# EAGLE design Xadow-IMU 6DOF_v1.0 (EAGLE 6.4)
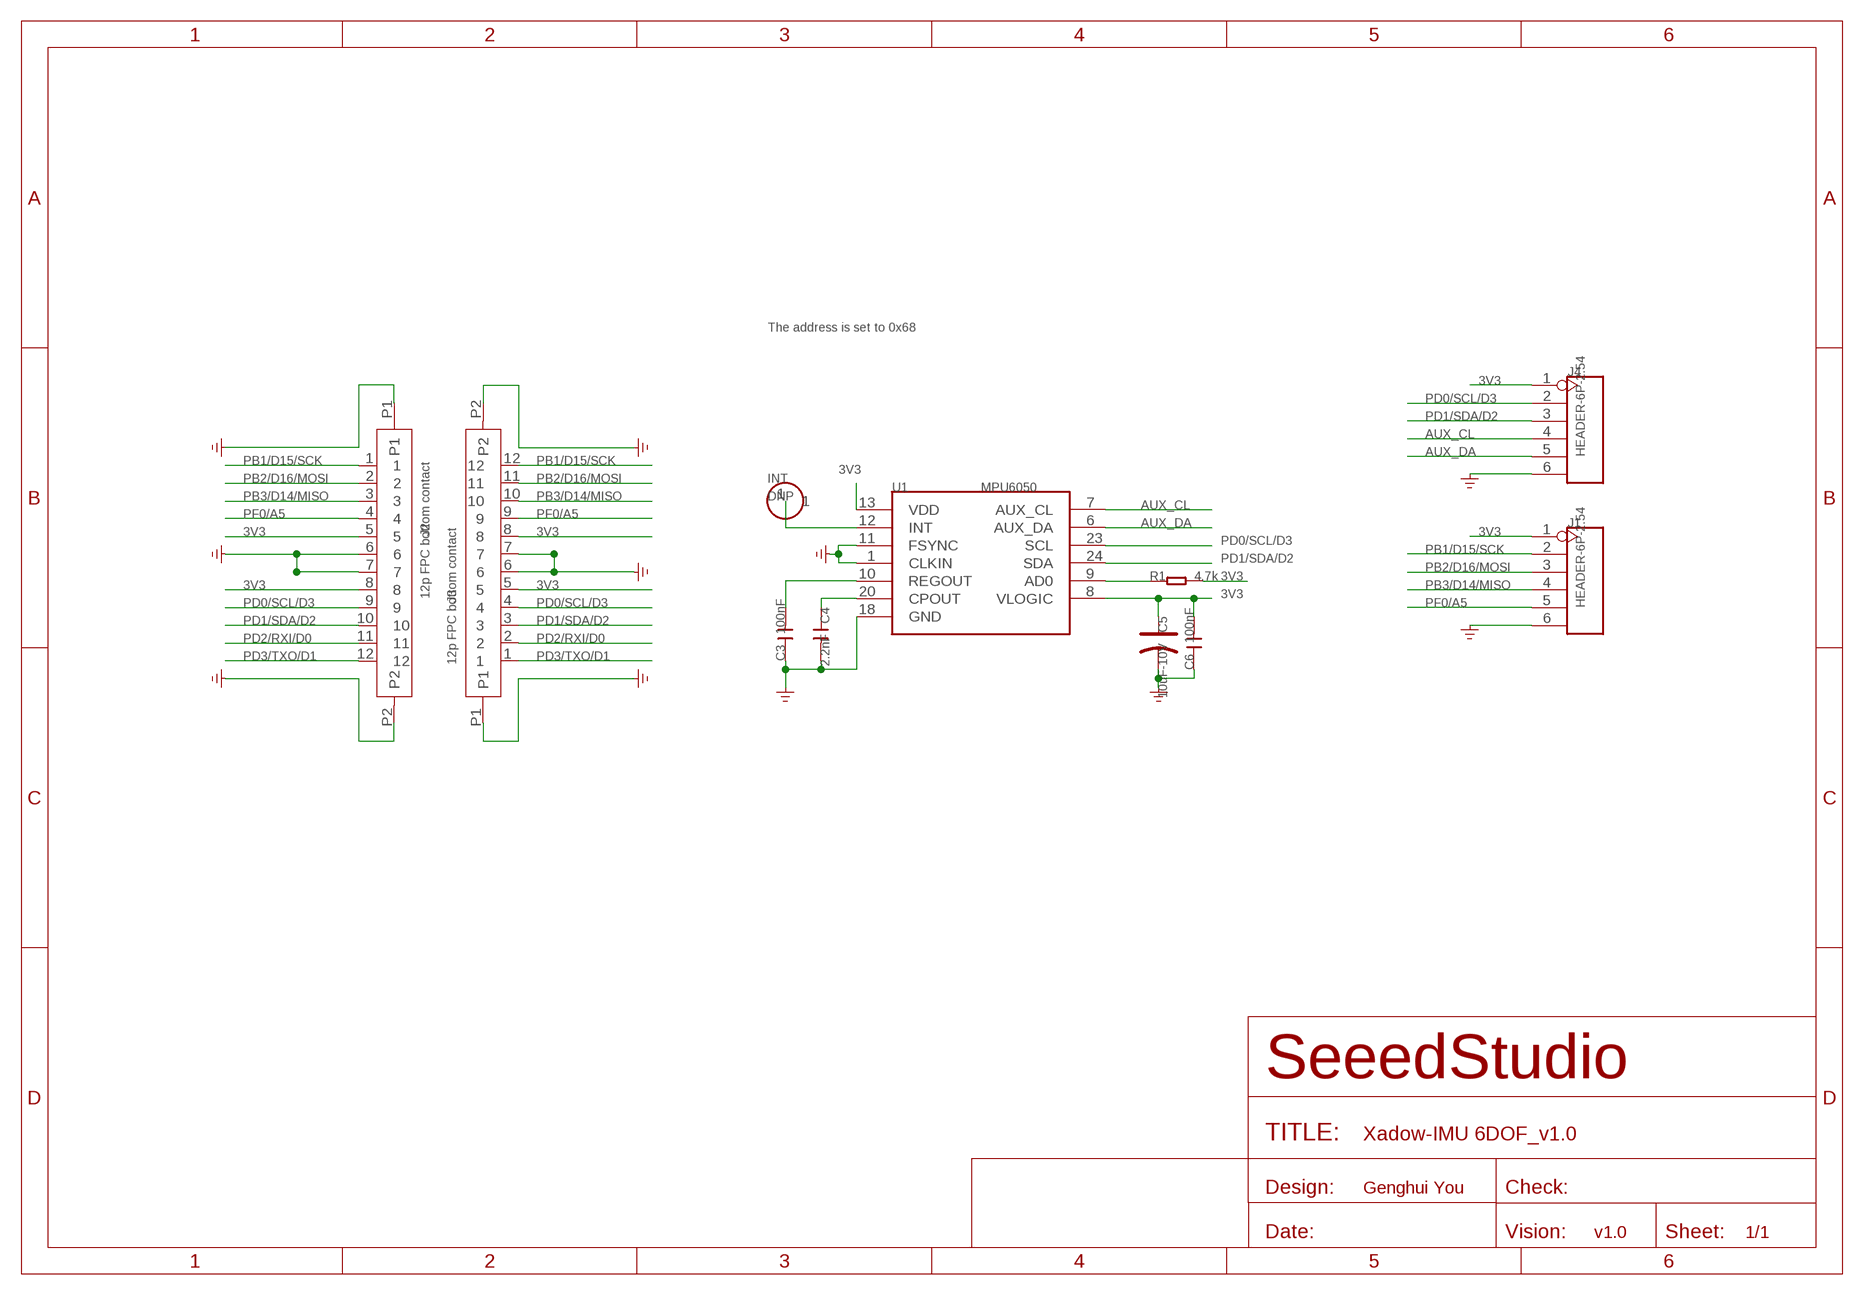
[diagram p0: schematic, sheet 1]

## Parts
C3  100nF  C-0603  [C0603]
C4  2.2nF  C-0603  [C0603]
C5  10uF-10V  CAP-AVX-A  [AVX-A]
C6  100nF  C-0603  [C0603]
INT  DNP  HEADER-1P-35  [1P-65/35MIL]
J1  HEADER-6P-2.54  HEADER-6P-65/35MIL  [6P-2.54-65/35MIL]
J2  12p FPC bottom contact  FPC052002-12LT  [12P-0.5]
J3  12p FPC bottom contact  FPC052002-12LT  [12P-0.5]
J4  HEADER-6P-2.54  HEADER-6P-65/35MIL  [6P-2.54-65/35MIL]
R1  4.7k  R-0603  [R0603]
U1  MPU6050  MPU-6050‘’  [QFN24]

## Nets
3V3: C5.+ C6.2 J1.1 J2.5 J2.8 J3.5 J3.8 J4.1 R1.2 U1.8(VLOGIC) U1.13(VDD)
AUX_CL: J4.4 U1.7(AUX_CL)
AUX_DA: J4.5 U1.6(AUX_DA)
GND: C3.1 C4.2 C5.- C6.1 J1.6 J2.6 J2.7 J2.P1 J2.P2 J3.6 J3.7 J3.P1 J3.P2 J4.6 U1.1(CLKIN) U1.11(FSYNC) U1.18(GND)
N$1: R1.1 U1.9(AD0)
N$21: INT.1 U1.12(INT)
N$22: C4.1 U1.20(CPOUT)
N$23: C3.2 U1.10(REGOUT)
PB1/D15/SCK: J1.2 J2.1 J3.12
PB2/D16/MOSI: J1.3 J2.2 J3.11
PB3/D14/MISO: J1.4 J2.3 J3.10
PD0/SCL/D3: J2.9 J3.4 J4.2 U1.23(SCL)
PD1/SDA/D2: J2.10 J3.3 J4.3 U1.24(SDA)
PD2/RXI/D0: J2.11 J3.2
PD3/TXO/D1: J2.12 J3.1
PF0/A5: J1.5 J2.4 J3.9

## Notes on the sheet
- The address is set to 0x68
- Genghui You
- v1.0

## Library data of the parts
C3 C4 C6 = Discrete:C*: Ceramic Capacitors
C5 = Discrete:CAP*: Electrolytic Capacitors,Tantalum Capacitors and Super Capacitors
INT = Connector :HEADER-1P
J1 J4 = Connector:HEADER-6P
J2 J3 = template:FPC052002-12LT
R1 = Discrete:R*
U1 = template:MPU-6050

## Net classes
0 default: width 0.152 mm, drill 0.305 mm, clearance 0.152 mm
1 GND: width 0.152 mm, drill 0.305 mm, clearance 0.152 mm to class 0, clearance 0.152 mm

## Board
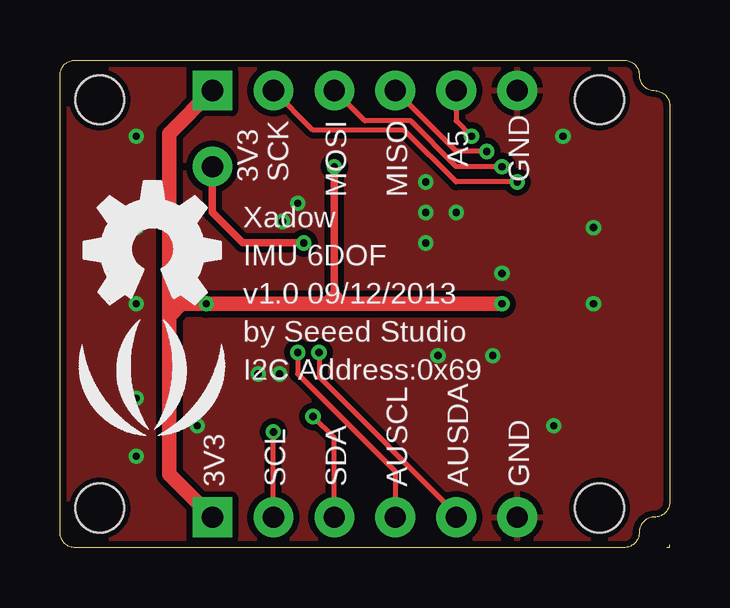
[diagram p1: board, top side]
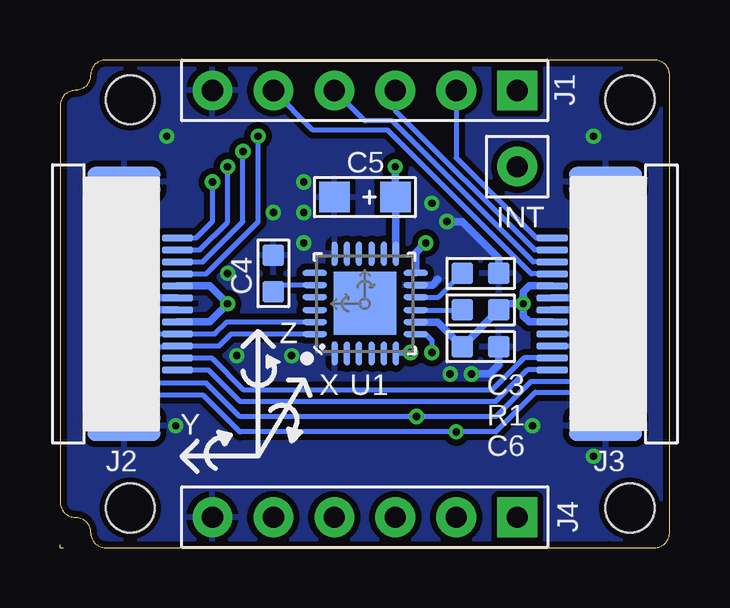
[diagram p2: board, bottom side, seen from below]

Size 25.4 x 20.32 mm. Coordinates in mm from the lower left corner, seen from the top.
Outline: 24.13,0.64 arc-90 24.77,1.27 arc90 25.4,1.91 25.4,18.42 arc90 24.77,19.05 arc-90 24.13,19.69 arc90 23.49,20.32 0.63,20.32 arc90 0,19.69 0,0.64 arc90 0.63,0 2.54,0 23.49,0 arc90 24.13,0.64
Outline: 24.13,0.64 24.13,0.64
Outline: 25.27,0 25.4,0 25.4,0.13
Copper layers (1*16): Top 0.035mm / dielectric 1.5mm / Bottom 0.035mm
Design rules "SeeedStudio_rule_no_angle_090911 *": minimum track width 6mil, minimum drill 12mil, track to track 6mil, track to pad 6mil, pad to pad 6mil, via to via 6mil, smd to smd 0mil, copper to edge 10mil, drill to drill 10mil, minimum pad ring 10mil, minimum via ring 6mil, stop-mask expansion 2mil, vias tented up to drill 100mil, thermal gap 10mil
Holes 2.03 mm at 22.48,1.65 22.48,18.67 1.65,18.67 1.65,1.65
tRestrict: 13 lines
bRestrict: area 20.3,10.1 to 21,10.2; area 4.5,10.1 to 5.1,10.2; area 13.4,9.3 to 14.4,9.4; 13 lines

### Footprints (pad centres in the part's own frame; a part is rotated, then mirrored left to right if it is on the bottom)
C0603 = smd 0.889 x 0.889: 1 -0.762,0; 2 0.762,0
AVX-A = smd 1.27 x 1.27: + -1.27,0; - 1.27,0
1P-65/35MIL = drill 0.889 pad 1.651: 1 0,0
6P-2.54-65/35MIL = drill 0.889 pad 1.651 square: 1 0,6.35 | drill 0.889 pad 1.651: 2 0,3.81; 3 0,1.27; 4 0,-1.27; 5 0,-3.81; 6 0,-6.35
12P-0.5 = smd 0.3 x 1.3: 1 -2.75,2.35; 2 -2.25,2.35; 3 -1.75,2.35; 4 -1.25,2.35; 5 -0.75,2.35; 6 -0.25,2.35; 7 0.25,2.35; 8 0.75,2.35; 9 1.25,2.35; 10 1.75,2.35; 11 2.25,2.35; 12 2.75,2.35 | smd 1.27 x 3.048: P1 -5.08,0.127; P2 5.08,0.127
R0603 = smd 0.889 x 0.889: 1 -0.762,0; 2 0.762,0
QFN24 = smd 1.016 x 0.254: 1 -2.066,1.257; 2 -2.066,0.75; 3 -2.066,0.247; 4 -2.066,-0.287; 5 -2.066,-0.792; 6 -2.066,-1.297; 13 2.086,-1.297; 14 2.086,-0.792; 15 2.086,-0.287; 16 2.086,0.247; 17 2.086,0.75; 18 2.086,1.257 | smd 0.254 x 1.016: 7 -1.267,-2.122; 8 -0.762,-2.122; 9 -0.258,-2.122; 10 0.278,-2.122; 11 0.78,-2.122; 12 1.287,-2.122; 19 1.287,2.082; 20 0.78,2.082; 21 0.278,2.082; 22 -0.258,2.082; 23 -0.762,2.082; 24 -1.267,2.082 | smd 2.616 x 2.616: P$1 0.02,-0.01

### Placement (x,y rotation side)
C3  7.87,11.43 180 bottom
C4  16.51,11.43 90 bottom
C5  12.7,14.61 180 bottom
C6  7.87,8.38 180 bottom
INT  6.35,15.88 0 bottom
J1  12.7,19.05 270 bottom
J2  22.86,10.16 270 bottom
J3  2.54,10.16 90 bottom
J4  12.7,1.27 270 bottom
R1  7.87,9.91 0 bottom
U1  12.7,10.16 90 bottom
U$2  [LOGO_SILK]  3.81,6.35 0 top
U$3  [OSHW_FILLX200_NOTEXT]  1.02,10.16 0 top

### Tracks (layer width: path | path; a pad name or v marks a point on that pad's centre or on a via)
3V3  (via drill 0.3 pad 0.64)
  Top 0.305: v11.43,15.88 11.43,10.67 | 11.43,10.67 11.43,10.29 11.56,10.16 | 11.43,10.67 11.94,10.16 | 11.43,10.67 11.05,10.29
  Top 0.61: J1.1 4.55,17.25 4.55,9.65 | 4.55,9.65 4.55,3.07 J4.1 | v18.41,10.16 11.94,10.16 11.56,10.16 v6.1,10.16 5.08,10.16 | 5.08,10.16 5.06,10.16 4.55,9.65 | 5.08,10.16 4.57,10.67
  Bottom 0.305: J2.5 19.16,10.91 v18.41,10.16 19.16,9.41 J2.8 | 11.4,14.71 11.43,14.73 C5.+ | U1.13 11.4,14.58 C5.+ | U1.8 9.65,9.4 C6.2 R1.2 7.11,10.03 6.98,10.16 v6.1,10.16 | J3.5 5.85,9.41 6.1,9.65 v6.1,10.16 | J3.8 5.85,10.91 6.1,10.67 v6.1,10.16 | C5.+ v11.43,15.88
AUX_CL  (via drill 0.3 pad 0.64)
  Top 0.203: v9.91,8.13 9.91,7.24 13.97,3.18 J4.4
  Bottom 0.203: U1.7 10.16,8.89 9.91,8.64 v9.91,8.13
AUX_DA  (via drill 0.3 pad 0.64)
  Top 0.203: v10.79,8.13 10.79,7.11 16.51,1.4 J4.5
  Bottom 0.203: U1.6 10.83,8.09 v10.79,8.13
GND  (via drill 0.3 pad 0.64)
  Bottom 0.305: J2.6 21.98,10.41 22.16,10.22 | 22.16,10.22 v22.23,10.16 | J2.7 21.85,9.91 22.16,10.22 | J3.7 3.42,10.41 v3.17,10.16 3.42,9.91 J3.6 | U1.11 9.89,10.94 9.65,11.18 | C3.1 7.11,12.07 8.64,13.59 v9.27,13.59 | C6.1 7.11,7.62 7.49,7.24 v8.25,7.24
  other vias: 18.41,11.43 16.51,13.97 15.24,13.97 15.24,15.24 15.24,12.7 15.75,8 9.14,7.24 9.91,14.35 3.17,13.34 3.17,6.22 3.17,17.15 3.17,3.81 22.23,13.34 20.95,17.15 20.57,5.08 5.71,5.08 18.03,8
  pour Bottom (isolate 0.254): 25.4,0 0,0 0,20.32 25.4,20.32
  pour Top (isolate 0.254): 25.4,0 0,0 0,20.32 25.4,20.32
N$1
  Bottom 0.203: U1.9 R1.1
N$21  (via drill 0.3 pad 0.64)
  Top 0.305: INT.1 6.35,13.97 7.62,12.7 v10.16,12.7
  Bottom 0.305: U1.12 10.58,12.28 v10.16,12.7
N$22
  Bottom 0.203: U1.20 16.24,10.94
  Bottom 0.305: 16.24,10.94 C4.1
N$23
  Bottom 0.203: U1.10 9.63,10.44 C3.2
PB1/D15/SCK  (via drill 0.3 pad 0.64)
  Top 0.203: v19.05,15.24 16.51,15.24 14.35,17.4 10.54,17.4 J1.2
  Bottom 0.203: J3.12 5.56,12.91 8.64,15.99 8.76,16.11 8.89,16.24 J1.2 | v19.05,15.24 19.05,13.59 19.73,12.91 J2.1
PB2/D16/MOSI  (via drill 0.3 pad 0.64)
  Top 0.203: v18.41,15.88 16.51,15.88 14.6,17.78 12.7,17.78 J1.3
  Bottom 0.203: J3.11 5.63,12.41 11.43,18.21 J1.3 | J2.2 19.57,12.41 18.41,13.56 v18.41,15.88
PB3/D14/MISO  (via drill 0.3 pad 0.64)
  Top 0.203: v17.78,16.51 16.51,16.51 J1.4
  Bottom 0.203: J3.10 5.69,11.91 11.56,17.78 12.7,17.78 J1.4 | J2.3 19.45,11.91 17.78,13.58 v17.78,16.51
PD0/SCL/D3  (via drill 0.3 pad 0.64)
  Top 0.203: J4.2 v8.89,4.83
  Bottom 0.203: J3.4 3.77,8.91 3.3,8.44 3.3,6.99 3.81,6.48 5.59,6.48 7.24,4.83 v8.89,4.83 17.91,4.83 19.43,6.35 21.64,6.35 22.1,6.81 22.1,8.44 21.62,8.91 J2.9 18.94,8.91 18.45,9.4 U1.23
PD1/SDA/D2  (via drill 0.3 pad 0.64)
  Top 0.203: J4.3 11.43,4.57 v10.54,5.46
  Bottom 0.203: J3.3 3.96,8.41 3.81,8.26 3.81,7.1 3.99,6.92 5.78,6.92 7.24,5.46 v10.54,5.46 17.91,5.46 19.3,6.86 21.41,6.86 21.59,7.04 21.59,8.2 21.41,8.38 20.54,8.38 J2.10 18.77,8.41 18.29,8.89 U1.24
PD2/RXI/D0
  Bottom 0.203: J2.11 19.09,7.91 17.76,6.58 7.39,6.58 6.06,7.91 J3.2
PD3/TXO/D1
  Bottom 0.203: J2.12 19.22,7.41 17.91,6.1 7.24,6.1 5.92,7.41 J3.1
PF0/A5  (via drill 0.3 pad 0.64)
  Top 0.203: J1.5 16.51,17.78 v17.14,17.15
  Bottom 0.203: J3.9 5.76,11.41 11.75,17.4 14.86,17.4 J1.5 | J2.4 19.31,11.41 17.14,13.58 v17.14,17.15

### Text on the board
tPlace: A5 | 3V3 | SCK | GND | MOSI | MISO | Xadow | IMU 6DOF | v1.0 09/12/2013 | by Seeed Studio | I2C Address:0x69 | 3V3 | SCL | SDA | AUSCL | AUSDA | GND
bPlace: Z | X | Y
tEnhance: Top Enhance 0.25~0.28mm
bEnhance: Bottom Enhance
bEnHoles: Holes on Bottom Enhance | All Holes are 70mil diameter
